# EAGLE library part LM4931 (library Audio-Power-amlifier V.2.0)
LM4931 Boomer™ Audio Power Amplifier Series Audio Subsystem with Mono High Efficiency Loudspeaker and Stereo Headphone Amplifiers
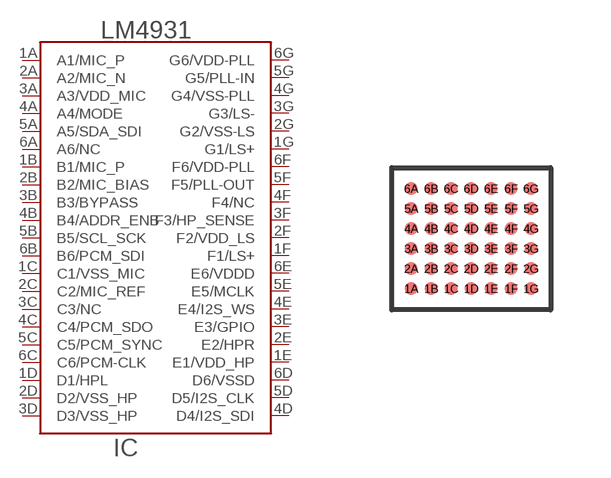
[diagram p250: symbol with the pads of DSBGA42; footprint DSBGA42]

Designator prefix IC

## LM4931  [DSBGA42]
1A  A1/MIC_P  in
1B  B1/MIC_P  in
1C  C1/VSS_MIC  pwr
1D  D1/HPL  out
1E  E1/VDD_HP  pwr
1F  F1/LS+  out
1G  G1/LS+  out
2A  A2/MIC_N  in
2B  B2/MIC_BIAS  out
2C  C2/MIC_REF  in
2D  D2/VSS_HP  pwr
2E  E2/HPR  out
2F  F2/VDD_LS  pwr
2G  G2/VSS-LS  pwr
3A  A3/VDD_MIC  pwr
3B  B3/BYPASS  in
3C  C3/NC  nc
3D  D3/VSS_HP  pwr
3E  E3/GPIO  out
3F  F3/HP_SENSE  in
3G  G3/LS-  out
4A  A4/MODE  in
4B  B4/ADDR_ENB  in
4C  C4/PCM_SDO  out
4D  D4/I2S_SDI  in
4E  E4/I2S_WS
4F  F4/NC  nc
4G  G4/VSS-PLL  pwr
5A  A5/SDA_SDI
5B  B5/SCL_SCK  in
5C  C5/PCM_SYNC
5D  D5/I2S_CLK
5E  E5/MCLK  in
5F  F5/PLL-OUT  out
5G  G5/PLL-IN  in
6A  A6/NC  nc
6B  B6/PCM_SDI  in
6C  C6/PCM-CLK
6D  D6/VSSD  pwr
6E  E6/VDDD  pwr
6F  F6/VDD-PLL  pwr
6G  G6/VDD-PLL  pwr

## Footprint DSBGA42 (pad centres in mm)
DSBGA42 www.ti.com
smd 0.32 x 0.32: 1A -1.5,-1.25; 1B -1,-1.25; 1C -0.5,-1.25; 1D 0,-1.25; 1E 0.5,-1.25; 1F 1,-1.25; 1G 1.5,-1.25; 2A -1.5,-0.75; 2B -1,-0.75; 2C -0.5,-0.75; 2D 0,-0.75; 2E 0.5,-0.75; 2F 1,-0.75; 2G 1.5,-0.75; 3A -1.5,-0.25; 3B -1,-0.25; 3C -0.5,-0.25; 3D 0,-0.25; 3E 0.5,-0.25; 3F 1,-0.25; 3G 1.5,-0.25; 4A -1.5,0.25; 4B -1,0.25; 4C -0.5,0.25; 4D 0,0.25; 4E 0.5,0.25; 4F 1,0.25; 4G 1.5,0.25; 5A -1.5,0.75; 5B -1,0.75; 5C -0.5,0.75; 5D 0,0.75; 5E 0.5,0.75; 5F 1,0.75; 5G 1.5,0.75; 6A -1.5,1.25; 6B -1,1.25; 6C -0.5,1.25; 6D 0,1.25; 6E 0.5,1.25; 6F 1,1.25; 6G 1.5,1.25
